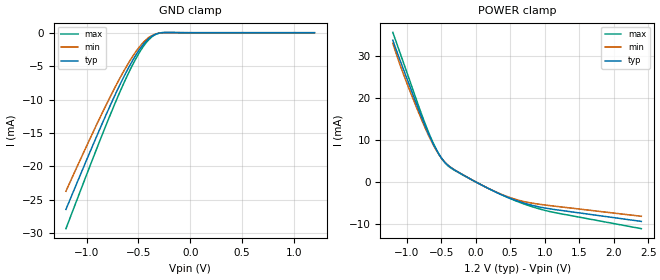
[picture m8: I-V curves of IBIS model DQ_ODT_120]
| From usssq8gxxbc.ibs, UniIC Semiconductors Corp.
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|   Model DQ_ODT_120
[Model] DQ_ODT_120
Model_type Input
Polarity   Non-Inverting
Enable   Active-High
Vinl =  8.300E-01
Vinh =  9.700E-01
C_comp   7.160E-13   7.131E-13   7.208E-13
C_comp_power_clamp   3.128E-13   3.125E-13   3.129E-13
C_comp_gnd_clamp   3.879E-13   3.847E-13   3.924E-13
[Model Spec]
Vinh   9.700E-01   9.250E-01   1.015E+00
Vinl   8.300E-01   7.850E-01   8.750E-01
[Temperature Range]   4.500E+01   9.500E+01   0.000E+00
[Voltage Range]   1.200E+00   1.140E+00   1.260E+00
[C Comp Corner]
C_comp_power_clamp   3.125E-13   3.129E-13   3.128E-13
C_comp_gnd_clamp   3.879E-13   3.847E-13   3.924E-13
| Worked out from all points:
|   GND clamp passes 1 mA (typ) near -0.41 V on its own axis
|   POWER clamp passes 1 mA (typ) near -0.11 V on its own axis
[GND_clamp]
|Voltage   I(typ)   I(min)   I(max)
-1.2V     -26.42mA   -23.7mA    -29.3mA
-875mV    -14.47mA   -12.81mA   -16.24mA
-750mV    -10.12mA   -8.886mA   -11.45mA
-650mV    -6.873mA   -5.975mA   -7.846mA
-575mV    -4.665mA   -4.008mA   -5.374mA
-500mV    -2.75mA    -2.321mA   -3.203mA
-425mV    -1.256mA   -1.034mA   -1.485mA
-375mV    -572uA     -467.3uA   -681.2uA
-325mV    -172.6uA   -148.9uA   -192.5uA
-250mV    14.61uA    2.428uA    39.85uA
1.2V      0A         0A         0A
[POWER_clamp]
|Voltage   I(typ)   I(min)   I(max)
-1.2V     33.62mA    32.92mA    35.5mA
-1.1V     29.1mA     28.02mA    30.83mA
-1V       24.73mA    23.61mA    26.17mA
-800mV    16.06mA    15.43mA    16.81mA
-675mV    11.11mA    10.8mA     11.48mA
-525mV    6.378mA    6.312mA    6.397mA
-450mV    4.717mA    4.723mA    4.648mA
-375mV    3.582mA    3.62mA     3.481mA
200mV     -1.701mA   -1.679mA   -1.687mA
650mV     -4.781mA   -4.472mA   -4.944mA
1.1V      -6.46mA    -5.684mA   -7.138mA
2.4V      -9.386mA   -8.17mA    -11.11mA
